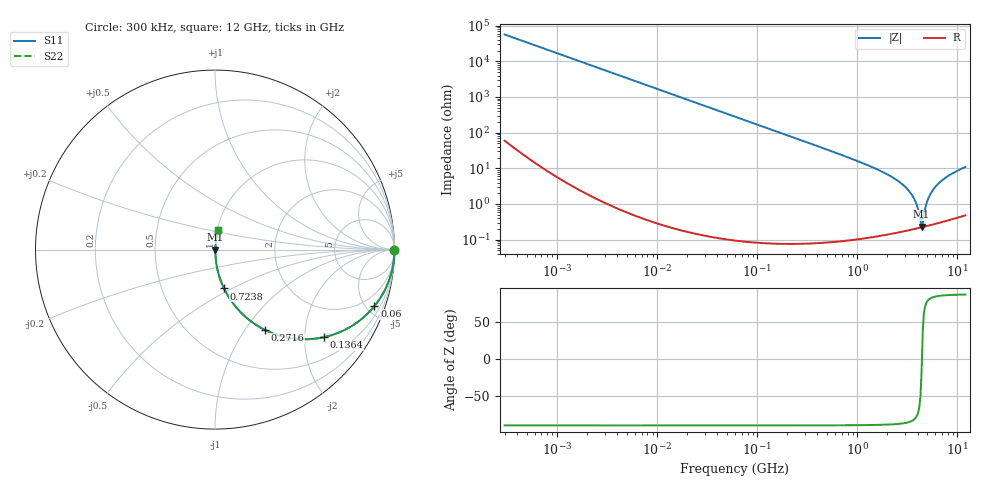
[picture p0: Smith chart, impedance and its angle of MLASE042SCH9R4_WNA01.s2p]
! MLASE042SCH9R4_WNA01  S-PARAMETER MODEL  ( General Type )
! Model Generated by TAIYO YUDEN Corporation (http://www.ty-top.com)
! Version 1.0
! TAIYO YUDEN Control No. 120810
! Copyright(c) 2012 TAIYO YUDEN CO.,LTD. All Rights Reserved.
! Product Description (link to TY-COMPAS)
! https://ds.yuden.co.jp/TYCOMPAS/or/detail?pn=MLASE042SCH9R4BWNA01&u=M
! Products Name : Multilayer Ceramic Capacitors
! Characteristics :
!  Capacitance : 9.4 pF , Rated Voltage : 16V , TCC : CH / C0H
!  Case Size : 0.4 x 0.2 / 0.016 x 0.008 [mm/inch] , Thickness : 0.2 / 0.008 [mm/inch]
!  (Conditions: Temperature = 25 degC , DC Bias Current/Voltage = 0A / 0V)
! External Node Assignments :
!  1  o---| |---o  2
! GND o---------o GND
! Frequency Range : 0.3MHz  -  12000MHz  [ 401 STEP ]
# MHz S RI R 50
! Freq[MHz].  S11 Real  S11 Imag  S21 Real  S21 Imag  S12 Real  S12 Imag  S22 Real  S22 Imag
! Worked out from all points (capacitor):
!   401 points, 300 kHz to 12 GHz, reference 50 ohm
!   read as one part in series: C = 9.39 pF near 316.3 kHz
!   lowest |Z| = 232 mohm at 4.385 GHz (marker M1)
!   series resonance near 4.416 GHz, so ESL is about 140 pH
!   S11 on the Smith chart (normalised r, x): 300 kHz: open; 60 MHz: 1.00, -5.65; 136.4 MHz: 1.00, -2.48; 271.6 MHz: 1.00, -1.24; 723.8 MHz: 1.00, -0.46; 12 GHz: 1.01, +0.22
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0.3  1 -0.00177  5e-06 0.00177  5e-06 0.00177  1 -0.00177
1.769972  0.9999 -0.0104  0.000111 0.0104  0.000111 0.0104  0.9999 -0.0104
10.44266  0.9962 -0.0614  0.00379 0.0614  0.00379 0.0614  0.9962 -0.0614
26.39317  0.9763 -0.152  0.0237 0.152  0.0237 0.152  0.9763 -0.152
60  0.8885 -0.3145  0.1115 0.3145  0.1115 0.3145  0.8885 -0.3145
136.3989  0.6065 -0.4882  0.3935 0.4882  0.3935 0.4882  0.6065 -0.4882
271.6094  0.279 -0.4479  0.721 0.4479  0.721 0.4479  0.279 -0.4479
353.9943  0.185 -0.3875  0.815 0.3875  0.815 0.3875  0.185 -0.3875
723.8279  0.0502 -0.2163  0.9498 0.2163  0.9498 0.2163  0.0502 -0.2163
2088.533  0.00537 -0.0626  0.9946 0.0626  0.9946 0.0626  0.00537 -0.0626
2795.104  0.00299 -0.0362  0.997 0.0362  0.997 0.0362  0.00299 -0.0362
3364.605  0.00232 -0.0211  0.9977 0.0211  0.9977 0.0211  0.00232 -0.0211
3740.715  0.00217 -0.0128  0.9978 0.0128  0.9978 0.0128  0.00217 -0.0128
3944.255  0.00215 -0.00874  0.9979 0.00874  0.9979 0.00874  0.00215 -0.00874
4270.516  0.00219 -0.00265  0.9978 0.00265  0.9978 0.00265  0.00219 -0.00265
4385.161  0.00222 -0.000633  0.9978 0.000633  0.9978 0.000633  0.00222 -0.000633
4623.766  0.00233 0.00453  0.9977 -0.00453  0.9977 -0.00453  0.00233 0.00453
4875.354  0.00248 0.0096  0.9975 -0.0096  0.9975 -0.0096  0.00248 0.0096
5140.631  0.0027 0.0146  0.9973 -0.0146  0.9973 -0.0146  0.0027 0.0146
6026.253  0.00371 0.0304  0.9963 -0.0304  0.9963 -0.0304  0.00371 0.0304
7854.144  0.00674 0.0576  0.9933 -0.0576  0.9933 -0.0576  0.00674 0.0576
12000  0.0164 0.107  0.9836 -0.107  0.9836 -0.107  0.0164 0.107
